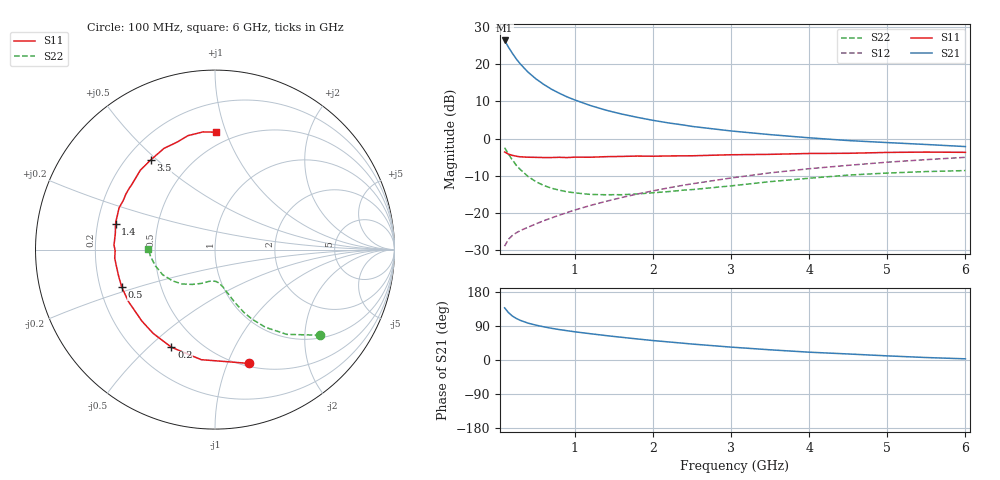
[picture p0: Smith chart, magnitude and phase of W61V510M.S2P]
! SIEMENS Small Signal Semiconductors
! BFR193W
! Si NPN RF Bipolar Junction Transistor in SOT323
! VCE = 1.5 V  IC = 10 mA
! Common Emitter S-Parameters:  September  1992
# GHz  S  MA  R  50
!  f  S11  S21  S12  S22
! GHz  MAG  ANG  MAG  ANG  MAG  ANG  MAG  ANG
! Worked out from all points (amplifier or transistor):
!   28 points, 100 MHz to 6 GHz, reference 50 ohm
!   highest |S21| = 26.4 dB at 100 MHz (marker M1)
!   |S21| within 3 dB of that: start of sweep to 185.6 MHz
!   unconditionally stable (mu >= 1): 928.4 MHz to 2.637 GHz
!   at 300 MHz: K = 0.57, MSG = 22.4 dB, |S12| = -24.7 dB
!   at 1.5 GHz: K = 1.05, MAG = 10.3 dB, |S12| = -16.3 dB
!   at 6 GHz: K = 0.92, MSG = 1.4 dB, |S12| = -5.0 dB
!   S11 on the Smith chart (normalised r, x): 100 MHz: 0.53, -1.19; 200 MHz: 0.35, -0.59; 500 MHz: 0.29, -0.18; 1.4 GHz: 0.28, +0.12; 3.5 GHz: 0.30, +0.48; 6 GHz: 0.40, +0.93
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0.1  0.6611 -73.5  20.9 137.6  0.0358 59.1  0.7564 -39.1
0.15  0.6181 -97.1  16.95 124.9  0.0445 52.1  0.6181 -49.8
0.2  0.5957 -114.1  14.01 115.9  0.0499 48.6  0.5164 -57.0
0.25  0.5802 -126.4  11.77 109.6  0.0542 47.0  0.438 -62.0
0.3  0.5698 -135.6  10.13 104.7  0.0579 47.2  0.3851 -65.3
0.4  0.5625 -149.0  7.832 97.3  0.0644 48.3  0.3095 -69.8
0.5  0.5601 -158.1  6.377 92.0  0.0713 50.5  0.264 -72.7
0.6  0.5568 -164.9  5.37 87.6  0.0786 52.5  0.2348 -75.7
0.7  0.557 -170.4  4.621 83.7  0.0858 54.4  0.2156 -77.6
0.8  0.5608 -175.1  4.079 80.3  0.0935 56.1  0.203 -79.9
0.9  0.5564 -179.2  3.641 77.3  0.1015 57.4  0.1925 -81.5
1  0.5633 177.3  3.309 74.4  0.1097 58.6  0.1867 -83.5
1.2  0.5624 170.9  2.784 69.3  0.1264 60.2  0.1776 -88.1
1.4  0.5722 165.6  2.411 64.4  0.1436 61.2  0.1759 -92.2
1.8  0.5829 156.5  1.932 55.5  0.18 61.8  0.1805 -100.8
2.2  0.5849 148.1  1.626 47.7  0.2178 61.2  0.194 -108.2
2.5  0.588 142.4  1.46 42.1  0.2469 60.1  0.2063 -113.6
3  0.607 133.3  1.268 34.0  0.2957 57.3  0.2316 -123.1
3.5  0.6147 125.6  1.132 26.9  0.3466 53.7  0.2641 -133.5
4.5  0.6351 109.4  0.942 15.9  0.4375 45.2  0.3234 -154.4
5.5  0.6591 95.8  0.834 6.5  0.522 36.1  0.3606 -173.8
6  0.6542 89.4  0.782 3.1  0.5608 31.2  0.3721 179.6
